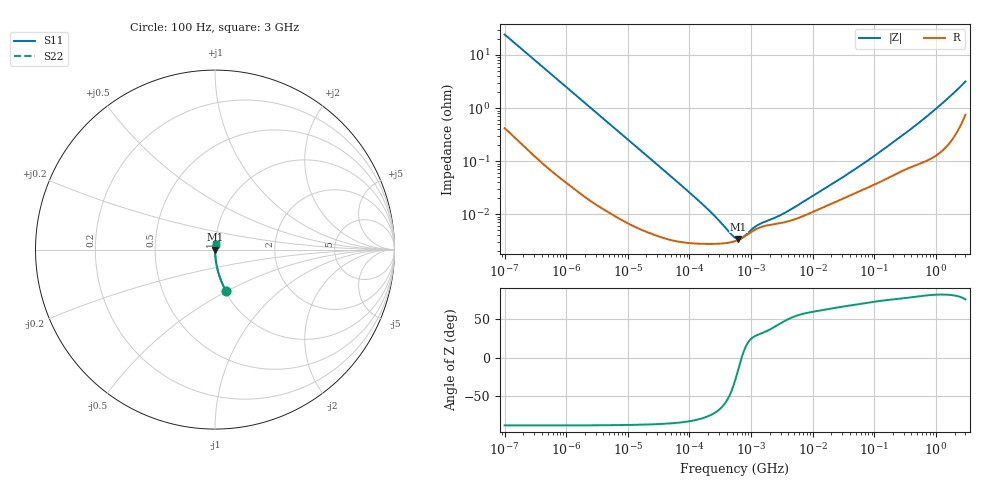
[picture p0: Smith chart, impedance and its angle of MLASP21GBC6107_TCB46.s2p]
! MLASP21GBC6107_TCB46  S-PARAMETER MODEL  ( Standard Model )
! Model Generated by TAIYO YUDEN Corporation (http://www.ty-top.com)
! Version 1.0
! TAIYO YUDEN Control No. 231201
! Copyright(c) 2023 TAIYO YUDEN CO.,LTD. All Rights Reserved.
! Product Description (link to TY-COMPAS)
! https://ds.yuden.co.jp/TYCOMPAS/or/detail?pn=MLASP21GBC6107MTCB46&u=M
! Products Name : Multilayer Ceramic Capacitors
! Characteristics :
!  Capacitance : 100 [uF] , Rated Voltage : 2.5 [V] , TCC : X6S
!  Case Size : 2.0 x 1.25 / 0.079 x 0.049 [mm/inch] , Thickness : 1.25 / 0.049 [mm/inch]
!  (Conditions: Temperature = 25 [degC] , DC Bias Voltage = 0 [V])
! External Node Assignments :
!  1  o---| |---o  2
! GND o---------o GND
! Frequency Range : 100Hz  -  3GHz  [ 401 STEP ]
# MHZ S RI R 50
! Freq[MHz].  S11 Real  S11 Imag  S21 Real  S21 Imag  S12 Real  S12 Imag  S22 Real  S22 Imag
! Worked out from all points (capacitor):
!   401 points, 100 Hz to 3 GHz, reference 50 ohm
!   read as one part in series: C = 65.1 uF near 109 Hz
!   lowest |Z| = 3.41 mohm at 623.2 kHz (marker M1)
!   series resonance near 703.5 kHz, so ESL is about 790 pH
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0.0001  0.0595 -0.2281  0.9405 0.2281  0.9405 0.2281  0.0595 -0.2281
0.000114  0.0471 -0.2035  0.9529 0.2035  0.9529 0.2035  0.0471 -0.2035
0.000199  0.0169 -0.121  0.9831 0.121  0.9831 0.121  0.0169 -0.121
0.000348  0.00605 -0.0703  0.9939 0.0703  0.9939 0.0703  0.00605 -0.0703
0.000724  0.0017 -0.0342  0.9983 0.0342  0.9983 0.0342  0.0017 -0.0342
0.001788  0.000429 -0.014  0.9996 0.014  0.9996 0.014  0.000429 -0.014
0.031977  3.87e-05 -0.000806  1 0.000806  1 0.000806  3.87e-05 -0.000806
0.102221  2.86e-05 -0.000249  1 0.000249  1 0.000249  2.86e-05 -0.000249
0.231582  2.76e-05 -0.000101  1 0.000101  1 0.000101  2.76e-05 -0.000101
0.263501  2.77e-05 -8.54e-05  1 8.54e-05  1 8.54e-05  2.77e-05 -8.54e-05
0.547723  3.11e-05 -1.84e-05  1 1.84e-05  1 1.84e-05  3.11e-05 -1.84e-05
0.623217  3.3e-05 -8.69e-06  1 8.69e-06  1 8.69e-06  3.3e-05 -8.69e-06
3.198641  6.92e-05 7.22e-05  0.9999 -7.22e-05  0.9999 -7.22e-05  6.92e-05 7.22e-05
4.323298  7.55e-05 9.54e-05  0.9999 -9.54e-05  0.9999 -9.54e-05  7.55e-05 9.54e-05
9.794414  0.000109 0.000189  0.9999 -0.000189  0.9999 -0.000189  0.000109 0.000189
50.26955  0.000255 0.000679  0.9997 -0.000679  0.9997 -0.000679  0.000255 0.000679
175.1444  0.0005 0.00195  0.9995 -0.00195  0.9995 -0.00195  0.0005 0.00195
396.7889  0.00079 0.004  0.9992 -0.004  0.9992 -0.004  0.00079 0.004
724.8677  0.00108 0.00702  0.9989 -0.00702  0.9989 -0.00702  0.00108 0.00702
1382.454  0.0019 0.0133  0.9981 -0.0133  0.9981 -0.0133  0.0019 0.0133
2752.553  0.00664 0.0276  0.9934 -0.0276  0.9934 -0.0276  0.00664 0.0276
3000  0.00834 0.0303  0.9917 -0.0303  0.9917 -0.0303  0.00834 0.0303
